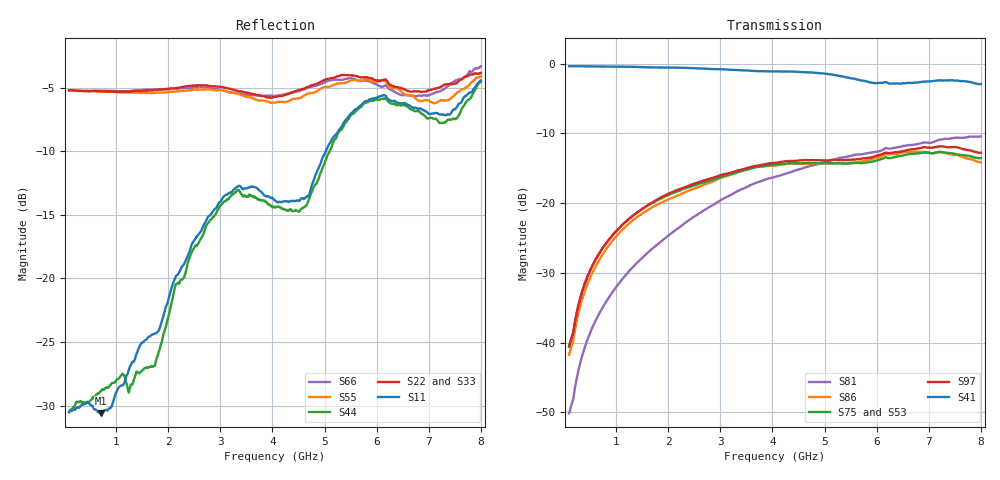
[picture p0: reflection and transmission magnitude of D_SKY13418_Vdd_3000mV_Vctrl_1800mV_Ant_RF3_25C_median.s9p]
# GHz S DB R 50
! THRU S21 mag phase subtraction.
! HALF_THRU
! EN33-165-011-v1_HALF_THRU_1 EN33-165-011-v1_HALF_THRU_2 EN33-165-011-v1_HALF_THRU_3 EN33-165-011-v1_HALF_THRU_4 EN33-165-011-v1_HALF_THRU_5 EN33-165-011-v1_HALF_THRU_6 EN33-165-011-v1_HALF_THRU_7 EN33-165-011-v1_HALF_THRU_8 EN33-165-011-v1_HALF_THRU_9
! THRU Ports: 1 2
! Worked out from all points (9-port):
!   801 points, 100 MHz to 8 GHz, reference 50 ohm
!   strongest paths, dB at 100 MHz, 2.075 GHz, 4.05 GHz, 6.025 GHz, 8 GHz:
!     S41: -0.4, -0.6, -1.1, -2.8, -2.9
!     S97: -40.5, -18.4, -14.2, -13.1, -12.7
!     S75: -40.6, -18.6, -14.5, -13.8, -13.5
!     S86: -41.7, -19.2, -14.6, -13.4, -14.1
!     S53: -41.0, -18.8, -14.6, -13.8, -13.6
!     S81: -50.1, -24.2, -16.2, -12.6, -10.4
!   lowest |S11| = -30.6 dB at 702.4 MHz (marker M1), VSWR 1.06, Z = 52.6 - j1.63 ohm
!   |S11| at or under -10 dB: start of sweep to 5.025 GHz
